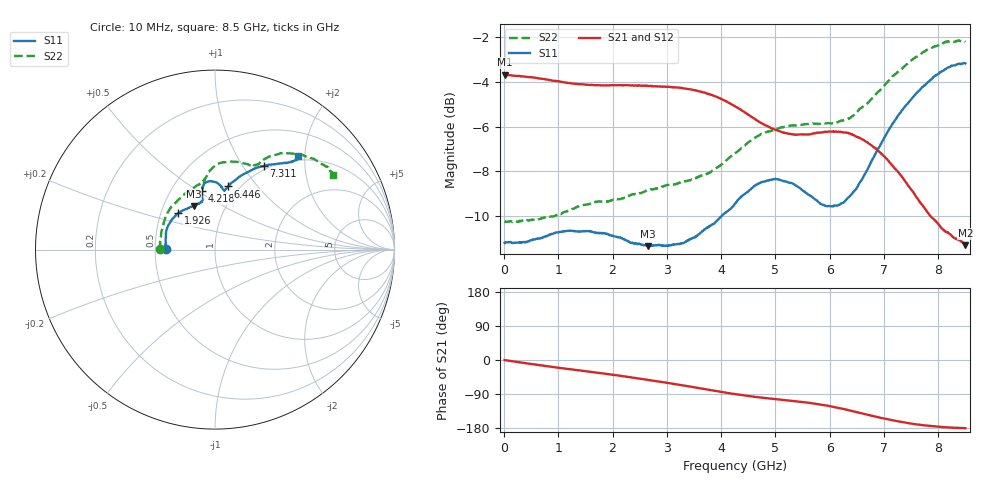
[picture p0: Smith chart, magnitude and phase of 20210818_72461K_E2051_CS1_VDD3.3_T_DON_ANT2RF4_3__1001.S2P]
!Agilent Technologies,E5071C,MY46417908,A.11.23
!Date: Wed Aug 18 14:33:55 2021
!Data & Calibration Information:
!Freq	S11:SOLT2(ON)	S21:SOLT2(ON)	S12:SOLT2(ON)	S22:SOLT2(ON)
!PortZ  Port1:50+j0  Port2:50+j0
!Above PortZ is port z conversion or system Z0 setting when saving the data.
!When reading, reference impedance value at option line is always used.
# Hz S dB R 50
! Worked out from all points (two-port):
!   1601 points, 10 MHz to 8.5 GHz, reference 50 ohm
!   highest |S21| = -3.66 dB at 10 MHz (marker M1); lowest = -11.3 dB at 8.5 GHz (marker M2)
!   |S21| within 3 dB of the highest: start of sweep to 6.666 GHz
!   lowest |S11| = -11.3 dB at 2.647 GHz (marker M3), VSWR 1.74, Z = 35.3 + j18.5 ohm
!   |S11| at or under -10 dB: start of sweep to 4.005 GHz
!   |S22| runs from -10.3 to -2.1 dB; largest |S21 - S12| = 0.0017
!   S11 on the Smith chart (normalised r, x): 10 MHz: 0.57, +0.00; 1.926 GHz: 0.61, +0.27; 4.218 GHz: 0.71, +0.52; 6.446 GHz: 0.89, +0.72; 7.311 GHz: 0.95, +1.25; 8.5 GHz: 0.93, +1.86
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1e7  -11.19 179.6  -3.66 -0.4  -3.66 -0.4  -10.23 179.8
5.671562e8  -11.04 168.4  -3.80 -11.8  -3.80 -11.8  -10.17 167.0
1.426769e9  -10.68 147.9  -4.09 -28.2  -4.10 -28.2  -9.51 143.3
1.925556e9  -10.82 135.5  -4.14 -37.4  -4.15 -37.4  -9.33 129.8
2.647206e9  -11.34 116.2  -4.17 -52.3  -4.17 -52.3  -8.85 111.9
2.843538e9  -11.30 112.4  -4.19 -56.6  -4.19 -56.6  -8.74 108.2
3.586412e9  -10.81 103.9  -4.41 -74.0  -4.40 -74.1  -8.23 99.6
3.910094e9  -10.23 103.5  -4.65 -81.9  -4.65 -81.9  -7.85 97.2
4.217856e9  -9.56 102.5  -5.03 -89.2  -5.03 -89.2  -7.25 94.6
4.255e9  -9.45 102.3  -5.08 -90.0  -5.07 -90.0  -7.19 94.2
4.631744e9  -8.61 99.6  -5.66 -97.5  -5.66 -97.5  -6.47 88.9
4.981956e9  -8.34 94.6  -6.12 -102.9  -6.12 -102.9  -6.13 81.8
5.671769e9  -9.13 83.8  -6.32 -113.9  -6.33 -113.9  -5.86 69.1
6.064431e9  -9.55 80.9  -6.22 -123.6  -6.23 -123.7  -5.84 65.8
6.446481e9  -8.89 78.3  -6.38 -135.9  -6.37 -136.0  -5.47 63.2
6.690569e9  -7.94 73.9  -6.69 -144.3  -6.68 -144.3  -4.96 62.0
7.088538e9  -6.13 64.8  -7.54 -157.2  -7.56 -157.3  -3.93 56.6
7.3114e9  -5.34 59.6  -8.18 -163.3  -8.18 -163.3  -3.44 52.9
7.571406e9  -4.57 54.0  -9.05 -169.2  -9.05 -169.3  -2.91 47.6
7.921619e9  -3.76 48.9  -10.16 -174.9  -10.14 -175.0  -2.41 40.3
8.128562e9  -3.42 47.8  -10.67 -177.4  -10.64 -177.4  -2.20 36.6
8.5e9  -3.16 48.3  -11.30 -179.8  -11.28 -179.9  -2.20 32.2
